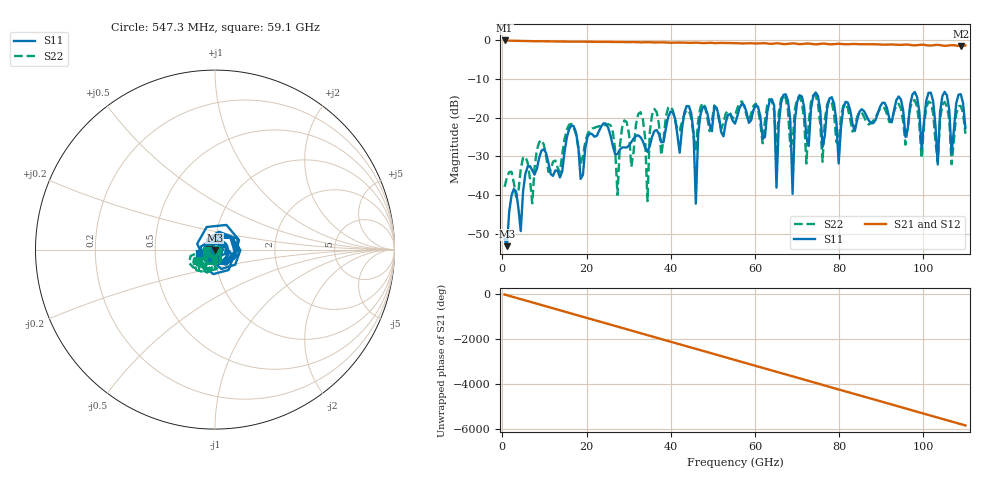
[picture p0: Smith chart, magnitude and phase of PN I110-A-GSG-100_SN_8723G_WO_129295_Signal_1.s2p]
!  2-Port S-parameters as saved by WinCal
!VAR DATE=03-13-2008  06:18:23
!VAR OPNAME=fvillan
# Hz S RI R 50.00
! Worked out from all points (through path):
!   201 points, 547.3 MHz to 110 GHz, reference 50 ohm
!   highest |S21| = -0.06 dB at 547.3 MHz (marker M1); lowest = -1.5 dB at 108.9 GHz (marker M2)
!   lowest |S11| = -53.2 dB at 1.095 GHz (marker M3), VSWR 1.00, Z = 49.8 - j0.134 ohm
!   |S11| at or under -10 dB: start of sweep to end of sweep
!   |S22| runs from -42.1 to -14.1 dB; largest |S21 - S12| = 0
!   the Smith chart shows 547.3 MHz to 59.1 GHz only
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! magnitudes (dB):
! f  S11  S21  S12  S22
! 547.3 MHz  -51.3  -0.1  -0.1  -37.8
! 1.095 GHz  -53.2  -0.1  -0.1  -35.4
! 19.15 GHz  -34.8  -0.4  -0.4  -29.8
! 27.36 GHz  -29.4  -0.4  -0.4  -39.9
! 32.84 GHz  -25.1  -0.5  -0.5  -18.6
! 34.48 GHz  -28.8  -0.5  -0.5  -41.5
! 37.21 GHz  -24.3  -0.6  -0.6  -21.8
! 44.33 GHz  -17.0  -0.7  -0.7  -18.2
! 45.97 GHz  -42.2  -0.6  -0.6  -28.1
! 47.61 GHz  -17.3  -0.7  -0.7  -16.2
! 55.27 GHz  -21.5  -0.7  -0.7  -19.6
! 64.03 GHz  -15.2  -0.9  -0.9  -15.7
! 65.12 GHz  -38.0  -0.8  -0.8  -28.4
! 67.31 GHz  -13.9  -1.0  -1.0  -15.0
! 68.96 GHz  -39.7  -0.8  -0.8  -26.4
! 70.05 GHz  -15.9  -0.9  -0.9  -15.1
! 72.24 GHz  -25.1  -0.9  -0.9  -31.8
! 73.88 GHz  -14.4  -1.0  -1.0  -14.2
! 76.07 GHz  -27.6  -0.9  -0.9  -31.4
! 91.94 GHz  -20.2  -1.1  -1.1  -21.2
! 108.9 GHz  -13.9  -1.5  -1.5  -17.0
! 110 GHz  -22.6  -1.4  -1.4  -24.1
